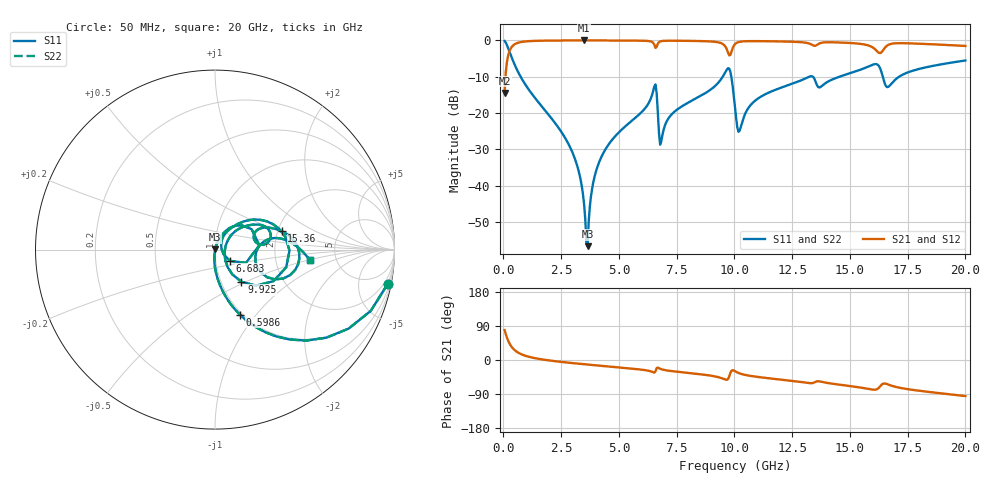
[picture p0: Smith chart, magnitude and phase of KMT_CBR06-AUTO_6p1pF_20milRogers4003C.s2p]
! Data measured by Modelithics Inc. support@modelithics.com 813-866-6335
! KEMET CBR06-AUTO 6.1pF, Pad Width= 0.851mm, Pad Length= 0.64mm, Pad Gap= 0.62mm, 20mil Rogers 4003C substrate Data, January 2022
# hz S ma R 50
! 2 Port Network Data from SP1.SP block
! freq  magS11  angS11  magS21  angS21  magS12  angS12  magS22  angS22
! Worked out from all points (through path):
!   401 points, 50 MHz to 20 GHz, reference 50 ohm
!   highest |S21| = -0.01 dB at 3.491 GHz (marker M1); lowest = -14.4 dB at 50 MHz (marker M2)
!   group delay of S21, straight-line fit = 14.7 ps
!   lowest |S11| = -56.6 dB at 3.641 GHz (marker M3), VSWR 1.00, Z = 50.1 + j0.0656 ohm
!   |S11| at or under -10 dB: 744.4 MHz to 9.492 GHz (8.747 GHz wide, 171 % of centre); 9.865 GHz to 13.23 GHz (3.368 GHz wide, 29.2 % of centre); 13.4 GHz to 14.54 GHz (1.146 GHz wide, 8.2 % of centre)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
!   |S22| runs from -56.6 to -0.2 dB; largest |S21 - S12| = 0
!   S11 on the Smith chart (normalised r, x): 50 MHz: 1, -10; 598.6 MHz: 0.97, -0.83; 6.683 GHz: 1.17, -0.15; 9.925 GHz: 1.25, -0.47; 15.36 GHz: 2.10, +0.50; 20 GHz: 3.16, -0.50
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5e7  0.9818 -11.1  0.1898 78.9  0.1898 78.9  0.9818 -11.1
2.495e8  0.7178 -44.9  0.6956 45.1  0.6956 45.1  0.7178 -44.9
5.98625e8  0.3877 -69.1  0.9212 20.8  0.9212 20.8  0.3877 -69.1
2.74325e9  0.04148 -95.2  0.998 -6.6  0.998 -6.6  0.04148 -95.2
3.391625e9  0.009874 -94.1  0.9987 -10.6  0.9987 -10.6  0.009874 -94.1
3.491375e9  0.005567 -89.4  0.9987 -11.1  0.9987 -11.1  0.005567 -89.4
3.641e9  0.001477 26.3  0.9987 -12.0  0.9987 -12.0  0.001477 26.3
3.94025e9  0.0132 71.0  0.9986 -13.7  0.9986 -13.7  0.0132 71.0
4.439e9  0.03266 71.2  0.998 -16.4  0.998 -16.4  0.03266 71.2
6.53375e9  0.2335 29.2  0.8701 -33.3  0.8701 -33.3  0.2335 29.2
6.683375e9  0.1032 -37.1  0.9006 -20.1  0.9006 -20.1  0.1032 -37.1
6.73325e9  0.05346 -27.8  0.9466 -21.7  0.9466 -21.7  0.05346 -27.8
9.4265e9  0.294 34.6  0.9161 -47.5  0.9161 -47.5  0.294 34.6
9.92525e9  0.2317 -50.6  0.7832 -26.8  0.7832 -26.8  0.2317 -50.6
1.0025e10  0.1202 -54.2  0.8891 -29.6  0.8891 -29.6  0.1202 -54.2
1.02245e10  0.05712 7.7  0.9572 -35.4  0.9572 -35.4  0.05712 7.7
1.10225e10  0.159 41.9  0.9779 -44.8  0.9779 -44.8  0.159 41.9
1.336662e10  0.321 14.3  0.8691 -61.1  0.8691 -61.1  0.321 14.3
1.536162e10  0.3855 15.4  0.9034 -71.8  0.9034 -71.8  0.3855 15.4
1.615962e10  0.4702 -10.0  0.7195 -77.4  0.7195 -77.4  0.4702 -10.0
1.670825e10  0.2361 0.6  0.8813 -65.8  0.8813 -65.8  0.2361 0.6
2e10  0.5296 -6.1  0.839 -95.2  0.839 -95.2  0.5296 -6.1
